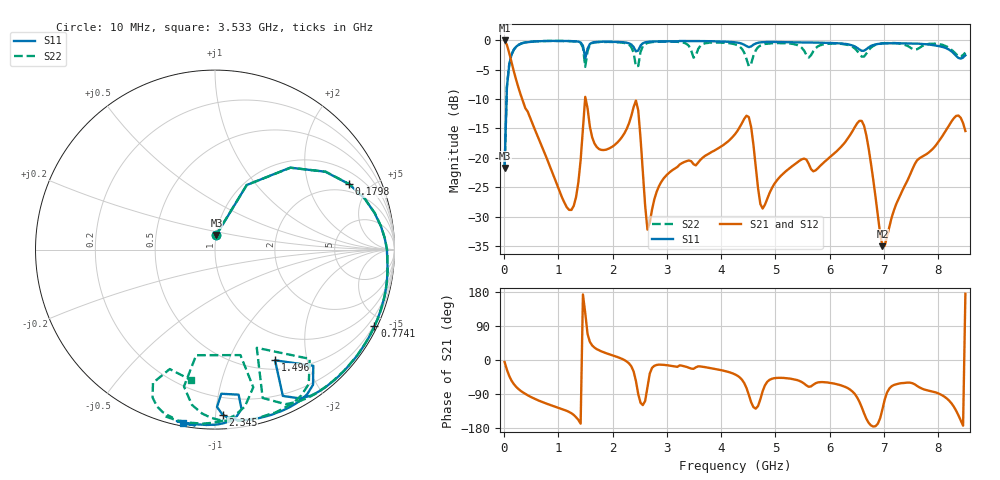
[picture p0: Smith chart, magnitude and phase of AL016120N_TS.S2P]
!AVX CORPORATION
!PART NUMBER AL016120N_TS
!DESCRIPTION: AIR CORE INDUCTOR, 120nH, 9 TURNS
!Agilent Technologies,E5071C,MY46102230,A.09.54
!Date: Mon Sep 03 16:38:16 2012
!Data & Calibration Information:
!Freq	S11:SOLT2(ON)	S21:SOLT2(ON)	S12:SOLT2(ON)	S22:SOLT2(ON)
# Hz S dB R 50
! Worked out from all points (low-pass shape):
!   201 points, 10 MHz to 8.5 GHz, reference 50 ohm
!   highest |S21| = -0.03 dB at 10 MHz (marker M1); lowest = -35.0 dB at 6.972 GHz (marker M2)
!   |S21| within 3 dB of the highest: start of sweep to 118.2 MHz
!   lowest |S11| = -21.7 dB at 10 MHz (marker M3), VSWR 1.18, Z = 50.1 + j8.25 ohm
!   |S11| at or under -10 dB: start of sweep to 46.1 MHz
!   |S22| runs from -21.6 to -0.1 dB; largest |S21 - S12| = 0.0036
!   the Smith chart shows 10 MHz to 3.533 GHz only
!   S11 on the Smith chart (normalised r, x): 10 MHz: 1.00, +0.17; 179.8 MHz: 1.57, +3.71; 774.1 MHz: 0.15, -4.39; 1.496 GHz: 0.62, -1.50; 2.345 GHz: 0.09, -1.04; 3.533 GHz: 0.01, -0.83
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1e7  -21.70 84.6  -0.03 -5.2  -0.04 -5.4  -21.60 85.1
5.245e7  -7.94 63.8  -0.79 -25.7  -0.78 -25.7  -7.94 63.8
1.798e8  -1.60 26.0  -5.27 -63.6  -5.26 -63.6  -1.58 25.9
7.741e8  -0.13 -25.7  -19.79 -114.7  -19.76 -114.8  -0.12 -27.0
1.24105e9  -0.14 -49.3  -28.84 -140.5  -28.84 -140.9  -0.17 -52.7
1.4533e9  -0.93 -65.1  -15.07 173.0  -15.07 172.9  -1.23 -72.2
1.49575e9  -3.08 -61.5  -9.62 124.0  -9.62 123.9  -4.52 -67.0
1.5382e9  -1.43 -49.8  -11.56 68.8  -11.55 68.8  -1.88 -49.1
1.75045e9  -0.26 -64.1  -18.50 25.6  -18.49 25.5  -0.32 -67.5
2.34475e9  -0.71 -87.4  -12.85 -16.7  -12.85 -16.8  -1.16 -98.4
2.4721e9  -1.73 -80.8  -11.92 -90.1  -11.92 -90.1  -4.37 -76.4
2.6419e9  -0.28 -87.1  -32.19 -71.3  -32.23 -71.6  -0.46 -86.1
2.85415e9  -0.19 -93.9  -24.81 -12.2  -24.80 -12.3  -0.24 -95.7
3.53335e9  -0.14 -100.4  -21.27 -19.4  -21.27 -19.4  -2.62 -100.2
4.255e9  -0.35 -111.1  -15.97 -38.0  -15.97 -38.0  -0.70 -126.4
4.5097e9  -1.17 -112.7  -13.06 -92.1  -13.07 -92.1  -4.42 -128.0
4.7644e9  -0.33 -114.8  -28.61 -82.3  -28.64 -82.5  -0.75 -121.5
5.6983e9  -0.41 -133.9  -22.29 -65.2  -22.28 -65.1  -1.86 -134.9
6.58975e9  -1.79 -151.0  -13.71 -124.6  -13.71 -124.6  -2.78 -151.9
6.9718e9  -0.56 -154.6  -35.00 -129.8  -34.93 -129.8  -0.51 -148.5
7.09915e9  -0.51 -157.7  -31.64 -75.2  -31.68 -75.3  -0.45 -151.2
8.5e9  -2.55 -174.4  -15.43 174.8  -15.43 174.8  -2.10 -151.1
